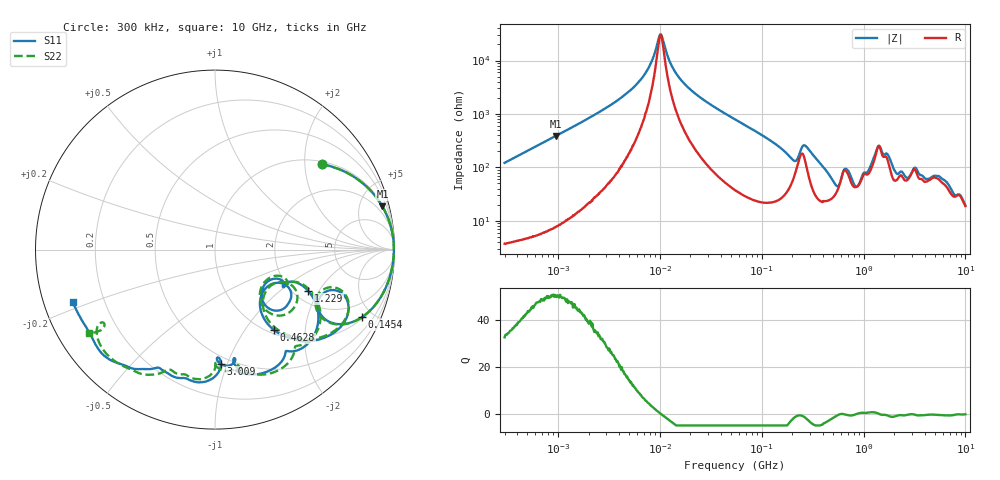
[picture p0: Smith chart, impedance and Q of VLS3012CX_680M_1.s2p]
! S-Parameter Data Generated by TDK Corporation
! Copyright(C) 2020 TDK Corporation.
! All Rights Reserved.
! TDK P/N: VLS3012CX-680M-1 (Inductor)
! Property: L=68uH at 1MHz
! Size(LxWxT): 3x3x1.2mm
! Model Type: s2p (Touchstone File Format Version 1.0)
! Frequency: DC=Yes Start=0.3MHz Stop=10000MHz 802points Log-sweep
! Model Generated on Aug. 18, 2020
! Port Assignments:
!  1 ---@@@--- 2
! Applicable Conditions:
!  Temperature = 25 degC
!  DC Bias Current = 0 A
!  Small Signal Operation
! Terms and conditions regarding TDK Simulation Models
! (1)This simulation model is being provided solely for informational purposes. Please refer to the specifications of the products in terms of detailed characteristics of such products.
! (2)In no event shall TDK Corporation of any of its subsidiaries be liable for any loss or damage arising, directly or indirectly,
!  From any information contained in this simulation model, including, but not limited to loss or damages arising from any inaccuracies, omissions or errors in connection with such information.
! (3)Any and all copyrights on this simulation model are owned by TDK Corporation.
!  Duplication or redistribution of this simulation model without prior written permission from TDK Corporation is prohibited.
! (4)This simulation model is subject to any modification or change without any prior notice.
! (5)Neither TDK Corporation nor any of its subsidiaries shall make any warranty, express or implied,
!  Including but not limited to the correctness, implied warranties of merchantability and fitness for a particular purpose with respect to this simulation models.
! (6)The use of this simulation model shall be deemed to have consented to the terms and conditions hereof.
# Hz S MA R 50
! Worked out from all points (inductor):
!   801 points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, 300 kHz to 10 GHz, reference 50 ohm
!   read as one part in series: L = 64.3 uH near 318.3 kHz
!   highest Q = 50.4 at 954.6 kHz (marker M1), where L = 64.4 uH
!   self-resonance near 10.15 MHz
!   S11 on the Smith chart (normalised r, x): 300 kHz: 1.07, +2.43; 145.4 MHz: 1.07, -4.33; 462.8 MHz: 1.06, -1.38; 1.229 GHz: 2.39, -1.61; 3.009 GHz: 0.44, -0.95; 10 GHz: 0.09, -0.18
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300000  0.7612 38.7  0.626 -49.5  0.6257 -49.5  0.7607 38.7
954628  0.9632 14.5  0.2495 -74.4  0.2495 -74.4  0.9633 14.4
1713600  0.9867 8.0  0.1401 -80.6  0.1401 -80.6  0.9868 8.0
5955893  0.9968 1.4  0.02745 -82.8  0.02744 -82.9  0.9968 1.4
9671944  0.9968 -0.1  0.004114 -39.2  0.004127 -39.4  0.9968 -0.1
1.03845e7  0.9967 -0.3  0.003338 13.8  0.003332 13.6  0.9967 -0.3
1.322782e7  0.9965 -1.1  0.01298 73.8  0.013 73.8  0.9965 -1.1
1.786051e7  0.996 -2.1  0.0284 80.7  0.02841 80.7  0.996 -2.1
5.477226e7  0.9863 -8.6  0.1244 78.7  0.1243 78.7  0.9863 -8.6
1.454054e8  0.902 -24.6  0.3549 59.9  0.3549 59.9  0.9009 -24.7
2.413764e8  0.7156 -18.6  0.3362 18.2  0.3362 18.2  0.7021 -17.5
3.126428e8  0.8126 -34.1  0.432 43.8  0.432 43.8  0.8109 -32.9
4.627802e8  0.5571 -53.7  0.6766 19.8  0.6766 19.8  0.5611 -52.1
5.911415e8  0.3664 -32.0  0.6438 -7.4  0.6436 -7.4  0.3788 -30.1
6.987102e8  0.5077 -37.6  0.5259 0.5  0.5259 0.5  0.5451 -38.5
8.872678e8  0.3387 -35.9  0.6721 -17.9  0.6721 -17.9  0.3297 -35.9
1.228555e9  0.567 -23.8  0.44 -45.6  0.4399 -45.6  0.5751 -23.2
1.403063e9  0.726 -39.8  0.2591 -34.9  0.259 -34.9  0.7272 -38.2
1.767019e9  0.7389 -64.5  0.3339 -9.8  0.3339 -9.8  0.7586 -60.8
3.008786e9  0.6366 -87.0  0.394 -49.5  0.3941 -49.5  0.6486 -89.7
6.333834e9  0.8337 -130.7  0.2592 -69.1  0.2589 -69.2  0.8246 -127.8
1e10  0.8455 -159.9  0.2223 -83.6  0.2217 -83.6  0.8413 -146.7
